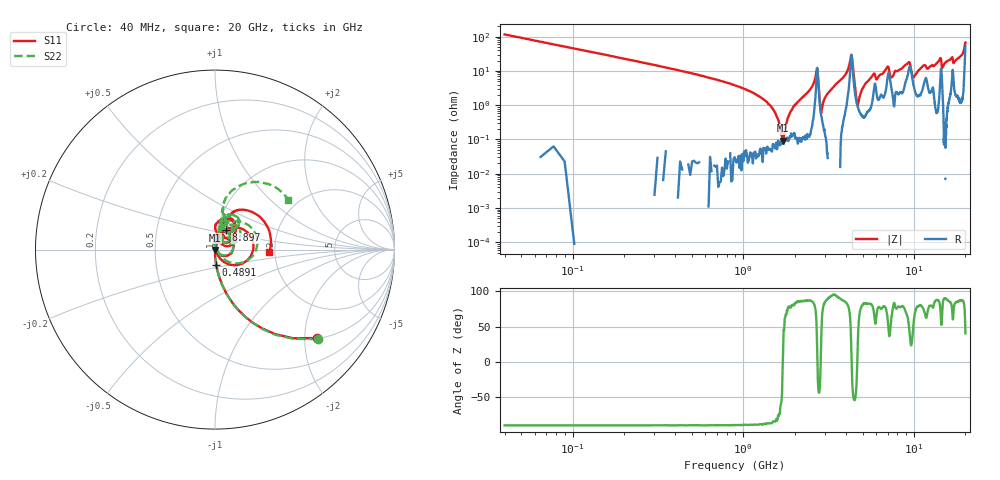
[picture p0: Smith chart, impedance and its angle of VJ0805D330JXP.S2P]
! VJ0805D330JXP
! DATE 10/29/2021  10:35
! CAPACITORS MOUNTED IN SERIES ON 25 MIL THICK MICROSTRIP SUBSTRATE
# GHz  S  MA  R  50.00
!  FREQ  S11M  S11A  S21M  S21A  S12M  S12A  S22M  S22A
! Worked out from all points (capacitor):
!   1601 points, 40 MHz to 20 GHz, reference 50 ohm
!   read as one part in series: C = 34.4 pF near 139.8 MHz
!   lowest |Z| = 91.7 mohm at 1.712 GHz (marker M1)
!   series resonance near 1.704 GHz, so ESL is about 250 pH
!   S11 on the Smith chart (normalised r, x): 40 MHz: 1.01, -2.30; 489.1 MHz: 1.00, -0.17; 8.897 GHz: 1.10, +0.24; 20 GHz: 1.86, -0.06
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0.04  0.7531 -40.9  0.6543 49.2  0.653 49.0  0.7601 -41.0
0.4891  0.08647 -85.3  0.9961 4.9  0.9953 4.9  0.08789 -85.2
1.399775  0.01257 -89.5  1 0.5  0.9991 0.5  0.0131 -83.4
1.71165  0.001781 -75.5  1 -0.1  0.9982 -0.1  0.002087 -50.8
2.647275  0.06062 67.6  0.982 -3.7  0.9808 -3.8  0.06176 71.9
2.90925  0.006702 51.8  0.9974 -0.7  0.9967 -0.7  0.006856 65.3
3.370825  0.02337 88.3  1.003 -2.3  1.003 -2.3  0.03029 99.2
4.269025  0.2059 27.4  0.822 -8.5  0.8212 -8.5  0.2322 35.5
4.718125  0.006617 29.3  0.9926 -0.7  0.9919 -0.7  0.01134 27.1
5.1797  0.03413 70.4  0.995 -2.6  0.9942 -2.6  0.0384 87.3
6.70165  0.08763 70.2  0.9791 -5.6  0.9781 -5.6  0.08857 74.3
7.40025  0.06033 58.6  0.9724 -3.7  0.9708 -3.7  0.05618 59.4
8.89725  0.1239 60.9  0.9496 -8.2  0.9476 -8.2  0.1471 65.1
10.02  0.05165 54.4  0.9692 -3.9  0.9673 -4.0  0.06395 53.3
11.42967  0.08154 57.7  0.9524 -8.2  0.9518 -8.2  0.1763 67.4
13.35083  0.1362 75.9  0.9815 -9.5  0.9807 -9.5  0.1355 79.5
14.2615  0.1867 59.1  0.9249 -13.3  0.9241 -13.3  0.2154 65.4
14.63575  0.08096 69.4  0.958 -7.6  0.9566 -7.6  0.1208 60.3
16.68165  0.194 66.2  0.9235 -14.6  0.9233 -14.6  0.2189 57.9
17.08085  0.1179 63.4  0.947 -10.6  0.9464 -10.7  0.1489 63.0
19.38873  0.2682 56.2  0.9242 -21.5  0.9225 -21.4  0.2761 79.3
20  0.3018 -2.7  0.6157 -19.8  0.6146 -19.8  0.4941 34.2
